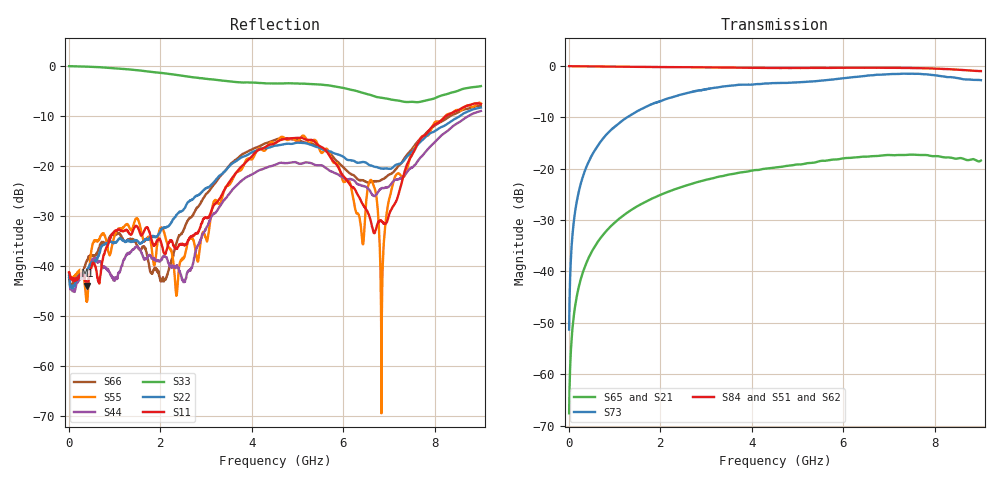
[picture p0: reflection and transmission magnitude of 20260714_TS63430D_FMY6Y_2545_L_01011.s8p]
# GHz S DB R 50
! CMT, SN0916, 25263762, 26.7.0
! Date: 15.07.2026 14:57:27
! Data: Format
! Freq S1.1:dB/Ang S1.2:dB/Ang S1.3:dB/Ang S1.4:dB/Ang S1.5:dB/Ang S1.6:dB/Ang S1.7:dB/Ang S1.8:dB/Ang
!  S2.1:dB/Ang S2.2:dB/Ang S2.3:dB/Ang S2.4:dB/Ang S2.5:dB/Ang S2.6:dB/Ang S2.7:dB/Ang S2.8:dB/Ang
!  S3.1:dB/Ang S3.2:dB/Ang S3.3:dB/Ang S3.4:dB/Ang S3.5:dB/Ang S3.6:dB/Ang S3.7:dB/Ang S3.8:dB/Ang
!  S4.1:dB/Ang S4.2:dB/Ang S4.3:dB/Ang S4.4:dB/Ang S4.5:dB/Ang S4.6:dB/Ang S4.7:dB/Ang S4.8:dB/Ang
!  S5.1:dB/Ang S5.2:dB/Ang S5.3:dB/Ang S5.4:dB/Ang S5.5:dB/Ang S5.6:dB/Ang S5.7:dB/Ang S5.8:dB/Ang
!  S6.1:dB/Ang S6.2:dB/Ang S6.3:dB/Ang S6.4:dB/Ang S6.5:dB/Ang S6.6:dB/Ang S6.7:dB/Ang S6.8:dB/Ang
!  S7.1:dB/Ang S7.2:dB/Ang S7.3:dB/Ang S7.4:dB/Ang S7.5:dB/Ang S7.6:dB/Ang S7.7:dB/Ang S7.8:dB/Ang
!  S8.1:dB/Ang S8.2:dB/Ang S8.3:dB/Ang S8.4:dB/Ang S8.5:dB/Ang S8.6:dB/Ang S8.7:dB/Ang S8.8:dB/Ang
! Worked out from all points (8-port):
!   2001 points, 10 MHz to 9 GHz, reference 50 ohm
!   strongest paths, dB at 10 MHz, 2.257 GHz, 4.505 GHz, 6.753 GHz, 9 GHz:
!     S84: -0.1, -0.3, -0.4, -0.4, -1.0
!     S51: -0.1, -0.2, -0.5, -0.4, -1.3
!     S62: -0.1, -0.3, -0.5, -0.4, -1.2
!     S73: -51.3, -6.1, -3.4, -1.7, -2.8
!     S65: -67.6, -24.2, -19.8, -17.5, -18.4
!     S21: -68.0, -24.2, -19.8, -17.5, -18.4
!   lowest |S11| = -43.9 dB at 410.1 MHz (marker M1), VSWR 1.01, Z = 50.3 - j0.58 ohm
!   |S11| at or under -10 dB: start of sweep to 8.236 GHz
